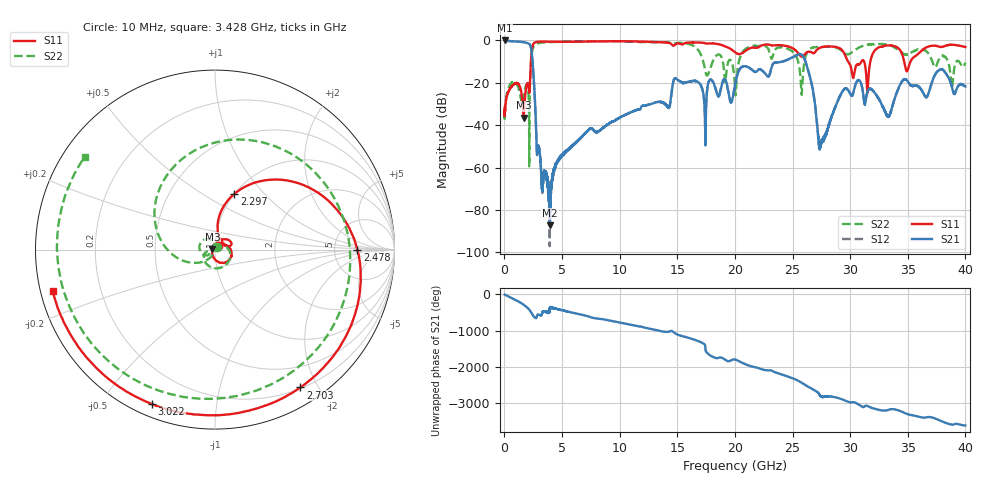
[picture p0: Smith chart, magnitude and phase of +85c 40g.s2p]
!Keysight Technologies,N5234A,MY52241180,A.10.60.03
!Date: Thursday, February 22, 2024 12:36:02
!Correction: S11(Full 2 Port(1,2))
!S21(Full 2 Port(1,2))
!S12(Full 2 Port(1,2))
!S22(Full 2 Port(1,2))
!S2P File: Measurements: S11, S21, S12, S22:
# Hz S  dB  R 50
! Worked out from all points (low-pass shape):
!   6401 points, 10 MHz to 40 GHz, reference 50 ohm
!   highest |S21| = -0.08 dB at 10 MHz (marker M1); lowest = -87.1 dB at 3.947 GHz (marker M2)
!   |S21| within 3 dB of the highest: start of sweep to 2.282 GHz
!   lowest |S11| = -36.4 dB at 1.66 GHz (marker M3), VSWR 1.03, Z = 48.6 + j0.393 ohm
!   |S11| at or under -10 dB: start of sweep to 2.293 GHz; 29.82 GHz to 30.98 GHz (1.168 GHz wide, 3.84 % of centre); 34.69 GHz to 35.23 GHz (547.4 MHz wide, 1.57 % of centre)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
!   |S22| runs from -59.4 to -0.4 dB; largest |S21 - S12| = 0.005
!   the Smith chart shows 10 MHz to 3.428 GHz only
!   S11 on the Smith chart (normalised r, x): 10 MHz: 1.03, +0.04; 2.297 GHz: 1.00, +0.70; 2.478 GHz: 8.68, -0.02; 2.703 GHz: 0.21, -1.78; 3.022 GHz: 0.05, -0.67; 3.428 GHz: 0.04, -0.12
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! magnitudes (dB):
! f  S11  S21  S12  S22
! 10 MHz  -31.7  -0.1  -0.1  -34.8
! 666.1 MHz  -21.5  -0.5  -0.5  -19.7
! 1.66 GHz  -36.4  -0.9  -0.9  -26.6
! 2.297 GHz  -9.7  -3.4  -3.4  -10.8
! 2.478 GHz  -2.0  -13.2  -13.2  -3.4
! 2.703 GHz  -0.9  -35.6  -35.6  -2.0
! 3.022 GHz  -0.6  -51.4  -51.5  -1.3
! 3.428 GHz  -0.6  -61.8  -63.4  -1.0
! 3.947 GHz  -0.7  -87.1  -79.9  -0.9
! 6.677 GHz  -0.6  -45.5  -45.6  -0.5
! 13.34 GHz  -0.9  -29.0  -29.0  -0.9
! 14.86 GHz  -1.9  -18.0  -18.0  -1.3
! 17.38 GHz  -1.3  -33.5  -33.5  -13.2
! 20 GHz  -5.6  -21.2  -21.2  -22.5
! 21.59 GHz  -3.5  -14.4  -14.4  -2.6
! 25.6 GHz  -6.8  -6.5  -6.5  -13.2
! 26.67 GHz  -5.7  -20.8  -20.8  -3.5
! 27.43 GHz  -3.4  -49.2  -49.1  -3.1
! 30.69 GHz  -11.3  -18.8  -18.7  -3.7
! 33.34 GHz  -2.4  -35.8  -35.8  -2.2
! 34.69 GHz  -10.1  -18.4  -18.4  -6.5
! 40 GHz  -3.2  -21.7  -21.7  -10.5
